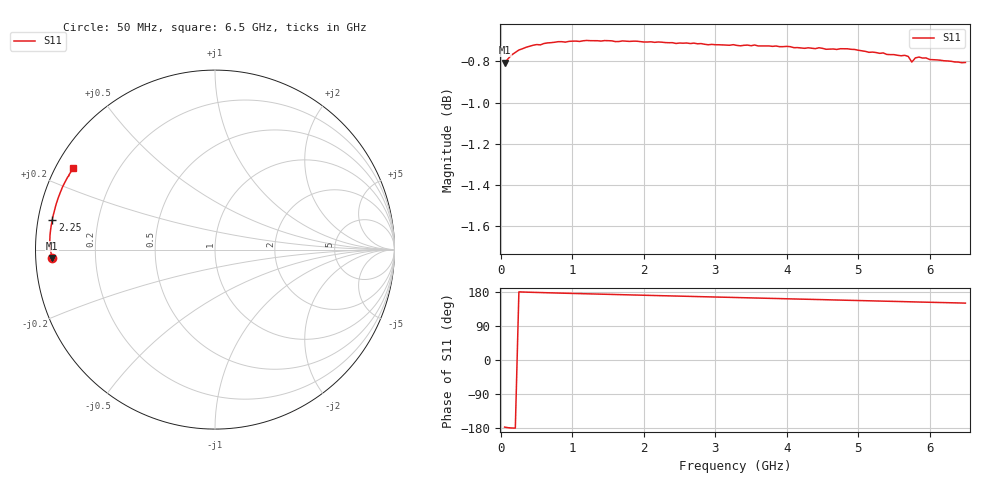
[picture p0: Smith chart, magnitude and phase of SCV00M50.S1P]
! Infineon Technologies  Discrete & RF Semiconductors
! BAR63-02L
! Si PIN Diode in TSLP-2
! IF = 0.5 mA
! S-Parameters:  March  2002
# GHz  S  MA  R  50
!  f  S11
! GHz  MAG  ANG
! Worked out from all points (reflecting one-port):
!   130 points, 50 MHz to 6.5 GHz, reference 50 ohm
!   lowest |S11| = -0.8 dB at 50 MHz (marker M1), VSWR 21.55, Z = 2.32 - j1.26 ohm
!   phase of S11 starts at -177 deg and turns -33 deg over the sweep
!   S11 on the Smith chart (normalised r, x): 50 MHz: 0.05, -0.03; 2.25 GHz: 0.04, +0.09; 6.5 GHz: 0.05, +0.27
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0.05  0.9113 -177.1
0.1  0.9134 -178.7
0.15  0.9154 -179.4
0.3  0.9185 179.4
0.45  0.9203 178.5
0.5  0.9206 178.3
0.75  0.9218 176.9
0.9  0.9219 176.2
1.15  0.9226 174.9
1.25  0.9226 174.5
1.4  0.9224 173.7
1.5  0.9226 173.3
1.7  0.9225 172.3
2.25  0.9219 169.7
2.5  0.9214 168.5
3.25  0.9206 165.1
3.3  0.9202 164.8
3.55  0.9204 163.7
4.1  0.9191 161.1
4.9  0.9182 157.4
5.1  0.9172 156.4
5.25  0.9165 155.8
5.45  0.9155 154.8
5.7  0.9145 153.7
5.75  0.9117 153.2
5.8  0.9138 153.2
5.85  0.9142 153.0
6.5  0.9115 150.1
